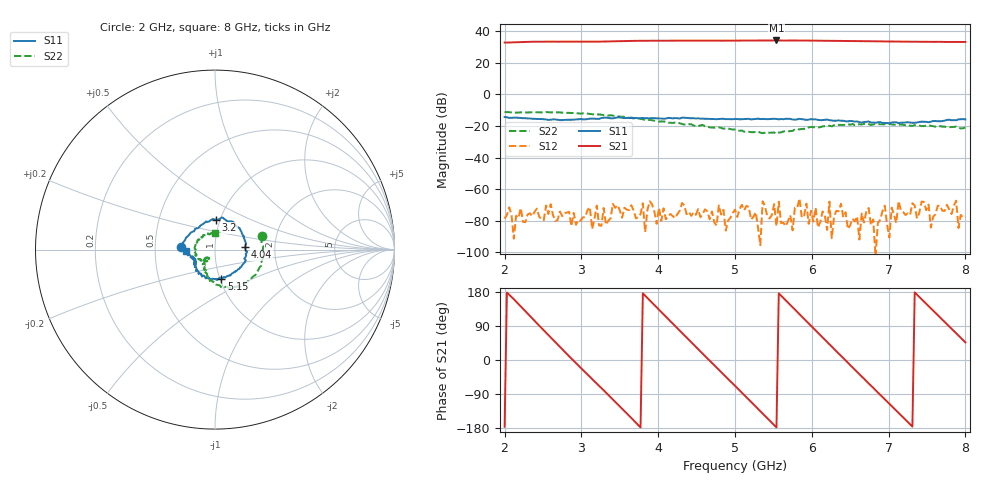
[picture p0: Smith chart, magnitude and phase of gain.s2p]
!Keysight Technologies,P5004A,MY58100454,A.15.10.06
!Date: Monday, July 24, 2023 16:07:35
!Correction: S11(Cdelta 2-Port  )
!S21(Cdelta 2-Port  )
!S12(Cdelta 2-Port  )
!S22(Cdelta 2-Port  )
!S2P File: Measurements: S11, S21, S12, S22:
# Hz S  dB  R 50
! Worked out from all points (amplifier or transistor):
!   201 points, 2 GHz to 8 GHz, reference 50 ohm
!   highest |S21| = 34.0 dB at 5.54 GHz (marker M1)
!   |S21| within 3 dB of that: start of sweep to end of sweep
!   unconditionally stable (mu >= 1): start of sweep to end of sweep
!   at 2.99 GHz: K = 99.91, MAG = 33.6 dB, |S12| = -80.0 dB
!   at 5 GHz: K = 43.20, MAG = 34.0 dB, |S12| = -72.9 dB
!   at 8 GHz: K = 81.94, MAG = 33.2 dB, |S12| = -77.6 dB
!   S11 on the Smith chart (normalised r, x): 2 GHz: 0.68, +0.02; 3.2 GHz: 0.96, +0.33; 4.04 GHz: 1.41, +0.04; 5.15 GHz: 1.02, -0.34; 8 GHz: 0.72, -0.01
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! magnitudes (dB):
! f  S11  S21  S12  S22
! 2 GHz  -14.4  32.7  -78.6  -11.3
! 3.02 GHz  -15.9  33.2  -77.8  -12.1
! 3.2 GHz  -15.6  33.3  -70.4  -12.8
! 4.01 GHz  -15.3  33.8  -71.8  -17.3
! 4.04 GHz  -15.4  33.8  -80.0  -17.2
! 5 GHz  -15.6  33.9  -72.9  -22.3
! 5.15 GHz  -15.6  34.0  -70.5  -23.7
! 5.33 GHz  -15.7  33.9  -95.4  -24.3
! 5.51 GHz  -15.5  34.0  -69.4  -24.2
! 5.54 GHz  -15.6  34.0  -83.4  -25.0
! 5.57 GHz  -15.9  34.0  -67.9  -24.2
! 5.6 GHz  -15.7  33.9  -81.4  -24.1
! 5.75 GHz  -16.0  34.0  -86.0  -23.2
! 5.84 GHz  -15.5  33.9  -65.8  -22.2
! 6.02 GHz  -15.9  33.9  -80.5  -20.9
! 6.2 GHz  -16.0  33.8  -85.7  -20.2
! 6.23 GHz  -16.4  33.8  -67.9  -19.9
! 6.26 GHz  -16.6  33.8  -91.0  -20.3
! 6.38 GHz  -16.7  33.7  -69.2  -19.4
! 7.01 GHz  -18.2  33.3  -90.6  -18.8
! 7.13 GHz  -18.2  33.3  -67.5  -19.3
! 8 GHz  -15.9  33.0  -77.6  -20.9
